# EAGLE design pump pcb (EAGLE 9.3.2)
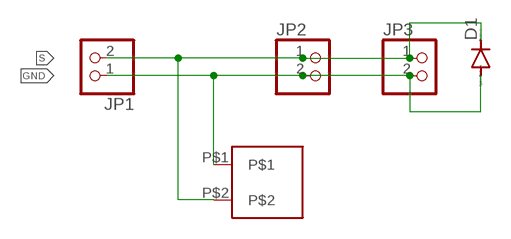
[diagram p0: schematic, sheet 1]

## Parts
D1  DIODE-SOD123  [SOD123]
JP1  PINHD-1X2  [1X02]
JP2  PINHD-1X2  [1X02]
JP3  PINHD-1X2  [1X02]
U$1  PUMP  [PUMP]

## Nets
GND: D1.A JP1.1 JP2.2 JP3.2 U$1.P$1
S: D1.C JP1.2 JP2.1 JP3.1 U$1.P$2

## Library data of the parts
D1 = diode:DIODE-: DIODE
JP1-JP3 = pinhead:PINHD-1X2: PIN HEADER
U$1 = pump:PUMP

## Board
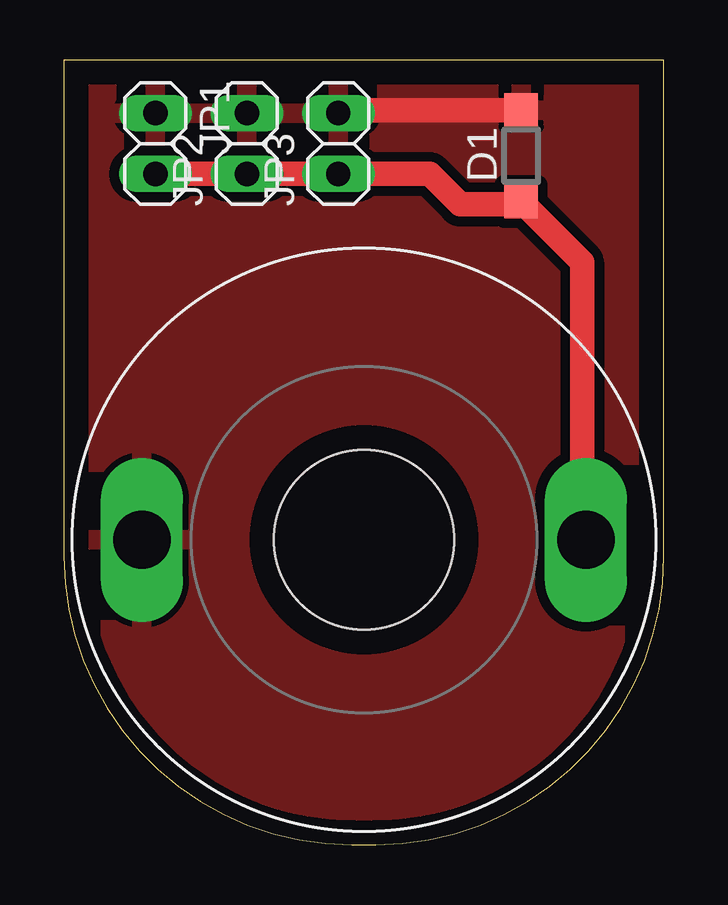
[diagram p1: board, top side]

Size 25 x 32.69 mm. Coordinates in mm from the lower left corner, seen from the top.
Outline: 0,32.69 0,12 arc90 12,0 13,0 arc90 25,12 25,32.69 0,32.69
Copper layers (1*16): Top 0.035mm / dielectric 1.5mm / Bottom 0.035mm
Design rules "default": minimum track width 6mil, minimum drill 0.35mm, track to track 6mil, track to pad 6mil, pad to pad 6mil, via to via 6mil, smd to smd 6mil, copper to edge 40mil, drill to drill 6mil, minimum pad ring 10mil, minimum via ring 8mil, stop-mask expansion 4mil, vias tented up to drill 0mil, thermal gap 10mil

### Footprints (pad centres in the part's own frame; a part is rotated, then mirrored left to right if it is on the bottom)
SOD123 = smd 1.4 x 1.4: A 1.9,0; C -1.9,0
1X02 = drill 1.016 long: 1 -1.27,0; 2 1.27,0
PUMP = drill 2.4 long: P$1 -9.25,0; P$2 9.25,0 | hole 7.5: 0,0

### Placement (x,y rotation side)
D1  19.05,28.7 90 top
JP1  3.81,29.21 270 top
JP2  7.62,29.21 90 top
JP3  11.43,29.21 90 top
U$1  12.5,12.7 0 top

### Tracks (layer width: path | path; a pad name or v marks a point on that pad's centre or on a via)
GND
  Top 1.016: D1.A 11.55,30.6 JP3.2
  pour Top (isolate 0.406): -1.27,41.91 -1.27,0 30.48,0 30.48,41.91
S
  Top 1.016: JP1.2 JP2.1 JP3.1 15.24,27.94 16.51,26.67 18.92,26.67 D1.C 21.59,24.26 21.59,12.86 U$1.P$2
